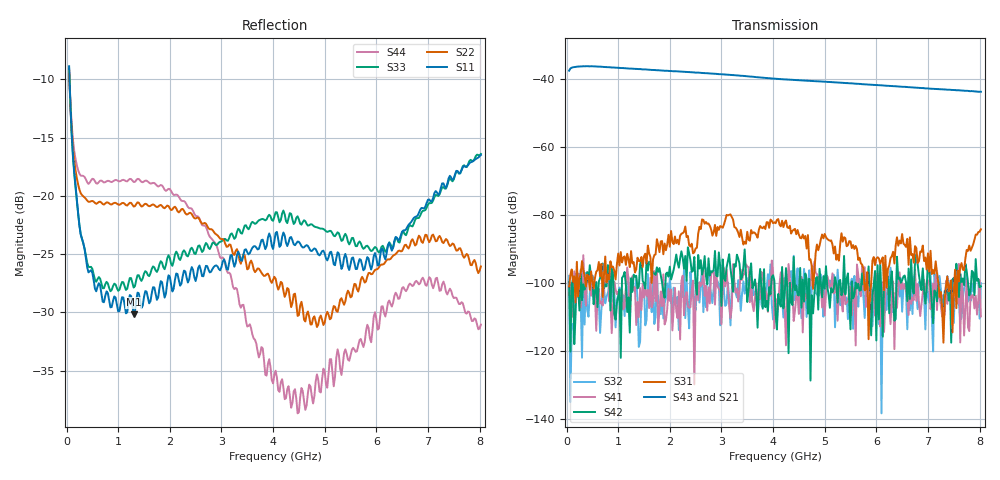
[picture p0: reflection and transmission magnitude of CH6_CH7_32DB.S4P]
!Agilent Technologies,E5071C,MY46316741,A.11.02
!Date: Mon Jun 01 10:35:18 2026
!Data & Calibration Information:
!1:CH6 INPUT 2:CH6 OUTPUT 3:CH7 INPUT 4:CH7 OUTPUT
!Freq	S11:SOLT4(ON)	S12:SOLT4(ON)	S13:SOLT4(ON)	S14:SOLT4(ON)
!	S21:SOLT4(ON)	S22:SOLT4(ON)	S23:SOLT4(ON)	S24:SOLT4(ON)
!	S31:SOLT4(ON)	S32:SOLT4(ON)	S33:SOLT4(ON)	S34:SOLT4(ON)
!	S41:SOLT4(ON)	S42:SOLT4(ON)	S43:SOLT4(ON)	S44:SOLT4(ON)
!PortZ  Port1:50+j0  Port2:50+j0  Port3:50+j0  Port4:50+j0
!Above PortZ is port z conversion or system Z0 setting when saving the data.
!When reading, reference impedance value at option line is always used.
# Hz S dB R 50
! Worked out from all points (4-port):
!   320 points, 50 MHz to 8.025 GHz, reference 50 ohm
!   strongest paths, dB at 50 MHz, 2.05 GHz, 4.05 GHz, 6.05 GHz, 8.025 GHz:
!     S43: -37.4, -37.5, -39.8, -41.7, -43.6
!     S21: -37.5, -37.6, -39.8, -41.7, -43.6
!     S31: -101.0, -87.8, -82.3, -92.7, -84.1
!     S42: -99.6, -97.5, -109.3, -110.6, -100.9
!     S41: -103.4, -113.9, -104.6, -108.6, -109.8
!     S32: -97.8, -111.6, -107.1, -112.0, -100.0
!   lowest |S11| = -30.2 dB at 1.3 GHz (marker M1), VSWR 1.06, Z = 47.5 - j1.76 ohm
!   |S11| at or under -10 dB: 58.7 MHz to end of sweep
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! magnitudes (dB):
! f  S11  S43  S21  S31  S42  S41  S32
! 50 MHz  -8.9  -37.4  -37.5  -101.0  -99.6  -103.4  -97.8
! 400 MHz  -26.1  -36.1  -36.2  -97.5  -96.7  -96.7  -107.7
! 1.3 GHz  -30.2  -36.9  -36.9  -93.8  -97.5  -102.1  -101.1
! 2.7 GHz  -26.0  -38.1  -38.2  -81.9  -97.8  -100.8  -107.0
! 4.475 GHz  -23.9  -40.2  -40.2  -84.3  -103.4  -103.4  -95.6
! 6.65 GHz  -22.4  -42.3  -42.2  -86.5  -104.6  -100.8  -108.0
! 8.025 GHz  -16.5  -43.6  -43.6  -84.1  -100.9  -109.8  -100.0
